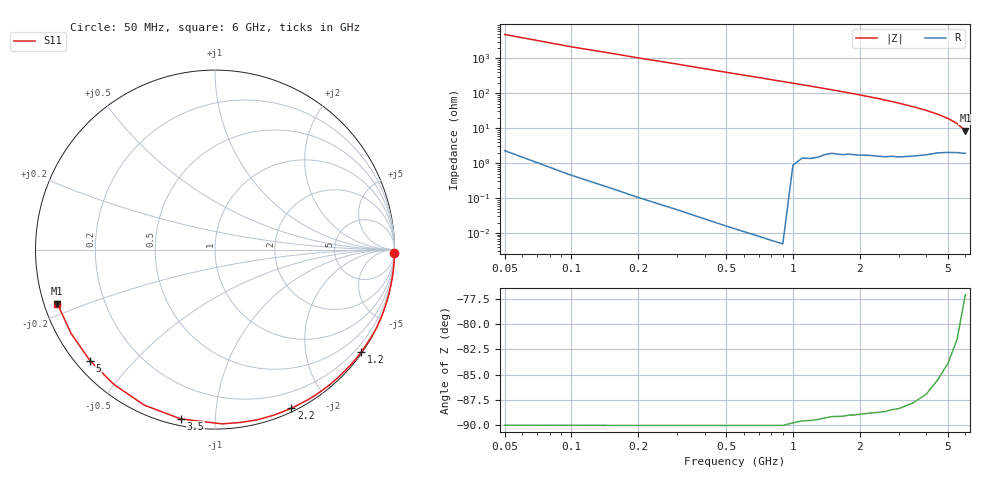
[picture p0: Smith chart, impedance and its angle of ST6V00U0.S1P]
! SIEMENS Discrete & RF Semiconductors
! BA892
! Si PIN Diode in SCD-80
! VR = 6 V
! S-Parameters:  September  1997
# GHz  S  MA  R  50
!  f  S11
! GHz  MAG  ANG
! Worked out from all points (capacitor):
!   34 points, 50 MHz to 6 GHz, reference 50 ohm
!   read as one part to ground: C = 750 fF near 50 MHz
!   lowest |Z| = 8.53 ohm at 6 GHz (marker M1)
!   S11 on the Smith chart (normalised r, x): 50 MHz: 0, -95; 1.2 GHz: 0.03, -3.18; 2.2 GHz: 0.03, -1.59; 3.5 GHz: 0.03, -0.82; 5 GHz: 0.04, -0.38; 6 GHz: 0.04, -0.17
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0.05  1 -1.2
0.15  1 -4.1
0.25  1 -7.0
0.4  1 -11.4
0.6  1 -17.3
0.7  1 -20.2
0.8  1 -23.2
0.9  1 -26.1
1  0.9978 -29.0
1.2  0.9951 -34.9
1.3  0.9937 -37.8
1.4  0.9915 -40.8
1.5  0.9895 -43.6
1.6  0.9888 -46.6
1.7  0.9878 -49.5
1.9  0.9852 -55.4
2  0.9839 -58.4
2.2  0.9812 -64.3
2.4  0.9792 -70.2
2.6  0.9771 -76.1
2.8  0.9734 -81.9
3  0.9715 -87.7
3.5  0.9624 -101.4
4  0.952 -114.5
4.5  0.939 -126.8
5  0.9315 -138.4
5.5  0.928 -149.8
6  0.9286 -161.1
